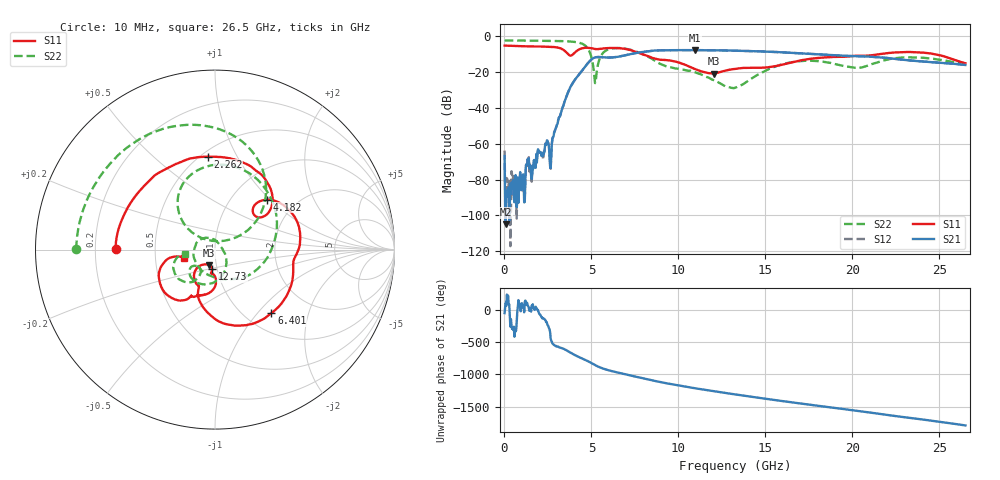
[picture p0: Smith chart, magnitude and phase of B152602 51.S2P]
!  2-Port S-parameters saved by WinCal
! VAR MeasName=S-Parameters (CALIBRATED_DATA) read from VNA (N5242A)
! VAR MeasDate=2016-1-5 16:33:23
! VAR NAME=B152602 51
! VAR FILENAME=B152602 51.S2P
! VAR DATE=2016-1-5 16:33:23
! VAR PHYS_PORTS=1,2
# Hz S DB R 50
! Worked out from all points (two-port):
!   801 points, 10 MHz to 26.5 GHz, reference 50 ohm
!   highest |S21| = -7.62 dB at 10.94 GHz (marker M1); lowest = -104.9 dB at 76.22 MHz (marker M2)
!   |S21| within 3 dB of the highest: 6.904 GHz to 19.04 GHz (12.14 GHz wide, 93.6 % of centre)
!   lowest |S11| = -20.8 dB at 12.03 GHz (marker M3), VSWR 1.20, Z = 46.2 - j7.99 ohm
!   |S11| at or under -10 dB: 3.671 GHz to 3.941 GHz (270.4 MHz wide, 7.1 % of centre); 7.975 GHz to 21.5 GHz (13.52 GHz wide, 91.8 % of centre); 24.76 GHz to end of sweep
!   |S22| runs from -28.9 to -2.2 dB; largest |S21 - S12| = 0.0031
!   S11 on the Smith chart (normalised r, x): 10 MHz: 0.29, +0.00; 2.262 GHz: 0.54, +0.77; 4.182 GHz: 1.44, +0.96; 6.401 GHz: 1.30, -1.19; 12.73 GHz: 0.94, -0.21; 26.5 GHz: 0.70, -0.07
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1e7  -5.13 179.5  -66.78 -52.1  -63.83 8.5  -2.24 179.8
7.6225e7  -5.14 177.0  -104.94 108.5  -85.51 -52.3  -2.24 178.8
1.755625e8  -5.16 173.0  -88.47 93.4  -80.32 89.8  -2.24 177.3
1.0696e9  -5.49 140.2  -77.14 47.6  -80.42 23.8  -2.30 163.4
2.26165e9  -5.69 94.5  -64.75 -137.0  -64.45 -137.8  -2.42 143.6
2.692112e9  -5.80 76.2  -66.39 -119.8  -65.72 -114.2  -2.46 135.3
3.4537e9  -7.96 37.7  -36.55 108.6  -36.56 108.8  -2.64 117.6
4.182175e9  -7.92 43.8  -22.58 1.5  -22.57 1.6  -3.28 92.4
4.447075e9  -6.68 29.9  -19.33 -30.7  -19.32 -30.6  -3.98 78.3
5.241775e9  -7.06 -7.0  -11.65 -139.1  -11.64 -139.0  -25.68 109.8
5.639125e9  -6.78 -18.3  -11.64 174.0  -11.64 174.2  -9.54 128.7
6.400712e9  -6.51 -48.4  -11.54 116.6  -11.52 116.7  -6.49 86.9
7.55965e9  -8.62 -93.2  -9.27 44.9  -9.23 45.0  -8.36 25.5
8.851038e9  -12.86 -113.3  -7.80 -31.3  -7.77 -31.4  -14.82 -65.7
1.093712e10  -18.14 -133.0  -7.62 -132.3  -7.63 -132.3  -19.97 147.4
1.202984e10  -20.76 -110.6  -7.77 -178.4  -7.77 -178.4  -24.39 102.3
1.27252e10  -19.08 -98.6  -7.84 153.0  -7.84 153.0  -27.97 60.2
1.3255e10  -18.16 -98.0  -7.97 132.3  -7.96 132.2  -28.72 22.9
1.577155e10  -16.22 -89.3  -8.78 36.6  -8.78 36.7  -16.11 -77.5
1.769208e10  -12.37 -96.8  -9.82 -32.3  -9.79 -32.1  -13.62 -124.5
2.209604e10  -9.25 -124.6  -12.19 171.3  -12.11 171.0  -12.77 -127.5
2.65e10  -14.97 -164.5  -15.94 12.4  -15.94 12.3  -15.51 -172.5
